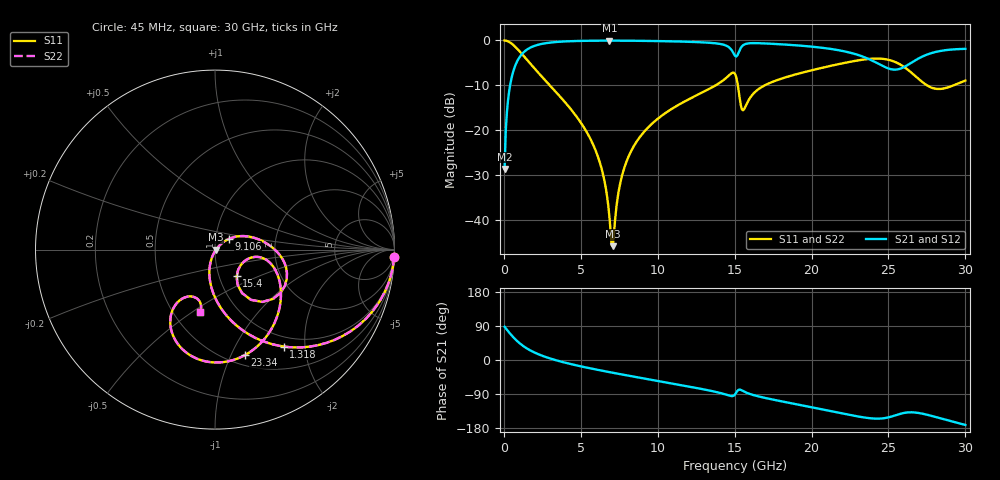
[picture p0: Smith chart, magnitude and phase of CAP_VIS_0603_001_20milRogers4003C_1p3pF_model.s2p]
! S-parameter model data by Modelithics Inc.  support@modelithics.com  813-866-6335  Tampa FL USA
! S-Parameter data specifications:
! Substrate: 20-mil Rogers 4003C, substrate thickness, H=0.508mm, Dielectric constant, Er=3.75
! PCB Mounting Pad Footprint: Pad width, PadW=0.90mm , Pad length, PadL=1.00mm , Pad gap, PadG (edge-to-edge)=1.00mm , Reference planes=3.0mm apart
! Created Wed Nov 18 13:18:07 2015
# hz S ma R 50
! 2 Port Network Data from SP1.SP block
! freq  magS11  angS11  magS21  angS21  magS12  angS12  magS22  angS22
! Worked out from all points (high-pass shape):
!   401 points, 45 MHz to 30 GHz, reference 50 ohm
!   highest |S21| = -0.05 dB at 6.86 GHz (marker M1); lowest = -28.5 dB at 45 MHz (marker M2)
!   |S21| within 3 dB of the highest: 1.167 GHz to 14.96 GHz (13.79 GHz wide, 171 % of centre); 15.21 GHz to 22.85 GHz (7.638 GHz wide, 40.1 % of centre)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
!   lowest |S11| = -45.7 dB at 7.084 GHz (marker M3), VSWR 1.01, Z = 50.5 - j0.13 ohm
!   |S11| at or under -10 dB: 2.989 GHz to 13.76 GHz (10.77 GHz wide, 129 % of centre); 15.21 GHz to 16.95 GHz (1.739 GHz wide, 10.8 % of centre); 27.51 GHz to 29.22 GHz (1.708 GHz wide, 6.02 % of centre)
!   |S22| runs from -45.7 to 0.0 dB; largest |S21 - S12| = 0
!   S11 on the Smith chart (normalised r, x): 45 MHz: 1, -49; 1.318 GHz: 0.84, -1.60; 9.106 GHz: 1.16, +0.14; 15.4 GHz: 1.21, -0.37; 23.34 GHz: 0.60, -1.13; 30 GHz: 0.67, -0.54
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4.5e7  0.9993 -2.4  0.03738 87.6  0.03738 87.6  0.9993 -2.4
2.696625e8  0.9756 -13.9  0.2187 76.0  0.2187 76.0  0.9756 -13.9
4.94325e8  0.9242 -24.7  0.3809 65.2  0.3809 65.2  0.9242 -24.7
1.318088e9  0.6615 -54.7  0.7481 35.1  0.7481 35.1  0.6615 -54.7
2.74095e9  0.3516 -82.0  0.9331 7.6  0.9331 7.6  0.3516 -82.0
5.062462e9  0.1176 -105.3  0.9886 -17.3  0.9886 -17.3  0.1176 -105.3
6.260662e9  0.04261 -111.2  0.994 -27.3  0.994 -27.3  0.04261 -111.2
6.859762e9  0.01096 -96.1  0.9946 -32.0  0.9946 -32.0  0.01096 -96.1
7.084425e9  0.005177 -14.4  0.9945 -33.7  0.9945 -33.7  0.005177 -14.4
7.458862e9  0.021 39.5  0.9941 -36.6  0.9941 -36.6  0.021 39.5
7.8333e9  0.03875 42.9  0.9934 -39.4  0.9934 -39.4  0.03875 42.9
9.106388e9  0.09628 37.7  0.9887 -48.8  0.9887 -48.8  0.09628 37.7
1.007992e10  0.1382 31.5  0.9831 -55.8  0.9831 -55.8  0.1382 31.5
1.374941e10  0.3157 2.7  0.9296 -84.0  0.9296 -84.0  0.3157 2.7
1.50225e10  0.4245 -40.3  0.6746 -91.1  0.6746 -91.1  0.4245 -40.3
1.539694e10  0.1918 -51.0  0.8249 -78.8  0.8249 -78.8  0.1918 -51.0
1.644536e10  0.2788 -10.5  0.9327 -95.0  0.9327 -95.0  0.2788 -10.5
2.003996e10  0.4675 -38.7  0.8521 -125.0  0.8521 -125.0  0.4675 -38.7
2.333501e10  0.6116 -74.4  0.6606 -151.2  0.6606 -151.2  0.6116 -74.4
2.505742e10  0.606 -102.8  0.4844 -150.8  0.4844 -150.8  0.606 -102.8
2.737894e10  0.3273 -123.6  0.6826 -143.2  0.6826 -143.2  0.3273 -123.6
3e10  0.3583 -103.3  0.8057 -171.4  0.8057 -171.4  0.3583 -103.3
